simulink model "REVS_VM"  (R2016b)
settings: Solver=ode3  StartTime=REVS.sim_start_time_secs  StopTime=Inf  FixedStep=REVS.sim_step_time_secs  MaxStep=REVS.sim_step_time_secs  EnableMultiTasking=on
StopFcn:
  | postproc_datalog;
  | postproc_audit;
  | postproc_result;
model workspace (MATLAB code in the model file):
  other statements: REVS_setup_variants
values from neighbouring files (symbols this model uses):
  accessory = class_accessory_data    [class_test_data.m]
  battery = class_battery_data    [class_accessory_data.m]    (also in class_REVS_electric.m = class_REVS_battery)
  brake = struct(	'max_torque_Nm',[], 						'proportion_norm',1.0, 						'inertia_kgm2',0.0)    [class_REVS_drive_axle.m]
  engine = class_engine_data    [class_test_data.m]
  final_drive = struct(	'gear_ratio',[], 								'efficiency_norm',[], 								'inertia_kgm2',[] )    [class_REVS_drive_axle.m]
  gear = class_REVS_gearbox    [class_REVS_AT_transmission.m]
  tire = struct(	'radius_m',[], 						'rolling_resistance_coefficient',0, 						'vehicle_weight_norm',1.0,  						'wheel_slip_torque_Nm',[],  						'inertia_kgm2',0.0)    [class_REVS_drive_axle.m]
  torque_converter = class_REVS_torque_converter    [class_REVS_AT_transmission.m]
  transmission = class_transmission_data    [class_test_data.m]
  vehicle = class_vehicle_data    [class_test_data.m]
undefined symbols (not defined in the file or in its folder): alternator, ambient, controls, convert, DelayTimeSecs, drive_cycle, driver, electric, gear_strategy, InitialCondition, InitialValue, LoadSource, LookupStructure, MultiplyPosInputs, Normalize, NumPhases, REVS, SpeedSource, starter, tableshift, UpperSaturationLimit, Value, VerboseLevel, VerboseSignal
libraries: simulink x153
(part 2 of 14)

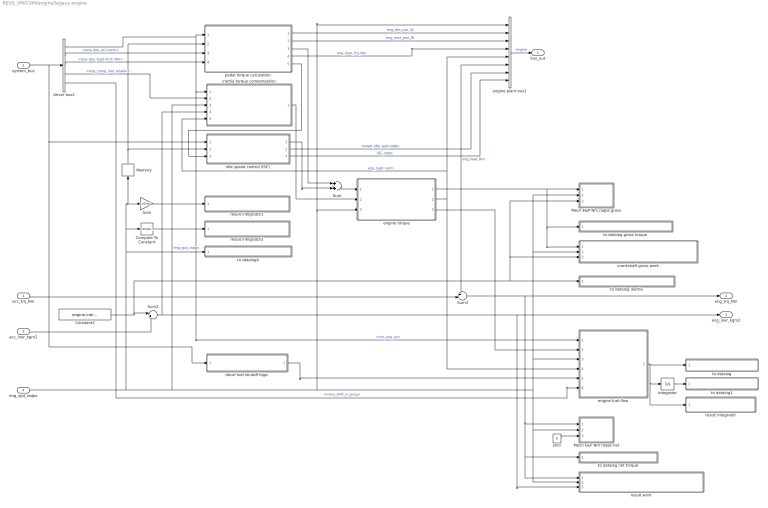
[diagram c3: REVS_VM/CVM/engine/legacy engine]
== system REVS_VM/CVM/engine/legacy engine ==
  system_bus : Inport
  acc_trq_Nm : Inport  Port=2
  acc_iner_kgm2 : Inport  Port=3
  eng_spd_radps : Inport  Port=4
  Compare To Constant : simulink/Logic and Bit Operations/Compare To Constant  relop=>  const=0  OutDataTypeStr=boolean  ZeroCross=off
  Constant2 : Constant  Value=engine.inertia_kgm2
  Gain : Gain  Gain=1/(2*pi)
  Integrator : Integrator
  Mech E&P Nm radps gross : Subsystem
  Mech E&P Nm radps net : Subsystem
  Memory : Memory
  Sum : Sum
  Sum2 : Sum  Inputs=|++
  Sum3 : Sum  Inputs=++|
  crankshaft gross work : Subsystem
  decel fuel shutoff logic : Subsystem
  driver bus2 : BusSelector  OutputSignals=powertrain.control.ctrl_eng_on,powertrain.trans.ctrl.eng_des_acl_norm,powertrain.trans.ctrl.eng_des_load_limit_Nm,powertrain.trans.ctrl.eng_comp_iner_enable,powertrain.trans.ctrl.core_ctl.trans_shift_in_prog
  engine fuel-flow : Subsystem
  engine plant bus1 : BusCreator  Inputs=8
  engine torque : Subsystem
  idle speed control (ISC) : Subsystem
  inertia torque compensation : Subsystem
  pedal torque calculation : Subsystem
  result integrator : Subsystem
  result integrator1 : Subsystem
  result integrator2 : Subsystem
  result work : Subsystem
  to datalog : Subsystem
  to datalog gross torque : Subsystem
  to datalog inertia : Subsystem
  to datalog net torque : Subsystem
  to datalog1 : Subsystem
  to datalog4 : Subsystem
  zero : Constant  Value=0
  bus_out : Outport
  eng_trq_Nm : Outport  Port=2
  eng_iner_kgm2 : Outport  Port=3
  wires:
  idle speed control (ISC)/3(ISC_state) -> engine plant bus1/8  "ISC_state"
  pedal torque calculation/5(current_min_trq_Nm) -> idle speed control (ISC)/3(eng_min_trq_Nm)
  Compare To Constant/1 -> result integrator2/1(in)
  Gain/1 -> result integrator1/1(in)
  driver bus2/5 -> engine fuel-flow/6(shift_in_prog)  "<trans_shift_in_prog>"
  Constant2/1 -> Sum2/1, crankshaft gross work/3(upstream_iner_kgm2), Mech E&P Nm radps gross/3(iner_kgm2), to datalog inertia/1(Var)
  zero/1 -> Mech E&P Nm radps net/3(iner_kgm2)
  eng_spd_radps/1 -> result work/2(speed_radps), Mech E&P Nm radps net/2(spd_radps), Mech E&P Nm radps gross/2(spd_radps), crankshaft gross work/2(speed_radps), engine fuel-flow/3(eng_spd_radps), engine torque/3(eng_spd_radps), engine plant bus1/1, inertia torque compensation/3(eng_spd_radps), to datalog4/1(Var), Compare To Constant/1, Gain/1, Memory/1  "eng_spd_radps"
  Sum3/1 -> eng_trq_Nm/1, Mech E&P Nm radps net/1(" trq_Nm"), to datalog net torque/1(Var), result work/1(torque_Nm)
  engine torque/1(eng_load_Nm) -> Mech E&P Nm radps gross/1(" trq_Nm"), to datalog gross torque/1(Var), crankshaft gross work/1(torque_Nm), Sum3/1, engine plant bus1/6  "eng_load_Nm"
  Integrator/1 -> to datalog1/1(Var)
  engine fuel-flow/1(fuel_flow_rate_gps) -> to datalog/1(Var), Integrator/1, result integrator/1(in)
  inertia torque compensation/1(comp_trq_Nm) -> engine torque/2(eng_fast_trq_Nm)
  pedal torque calculation/4(current_max_trq_Nm) -> engine plant bus1/4  "eng_max_trq_Nm"
  driver bus2/3 -> pedal torque calculation/4(eng_des_load_limit_Nm)  "<eng_des_load_limit_Nm>"
  driver bus2/4 -> inertia torque compensation/2(comp_iner_enable)  "<eng_comp_iner_enable>"
  Sum2/1 -> inertia torque compensation/4(iner_kgm2), eng_iner_kgm2/1, result work/3(upstream_iner_kgm2)
  engine torque/2(eng_load_norm) -> inertia torque compensation/5(load_norm), engine plant bus1/5, engine fuel-flow/4(eng_load_norm)  "eng_load_norm"
  Memory/1 -> idle speed control (ISC)/2(eng_spd_radps), pedal torque calculation/2(eng_spd_radps)
  driver bus2/1 -> pedal torque calculation/1(eng_on), engine fuel-flow/1(eng_on), inertia torque compensation/1(eng_on)  "<ctrl_eng_on>"
  system_bus/1 -> driver bus2/1, idle speed control (ISC)/1(system_bus), decel fuel shutoff logic/1(system_bus)
  Sum/1 -> engine torque/1(eng_slow_trq_Nm)
  idle speed control (ISC)/1(trq_out_Nm) -> Sum/2
  pedal torque calculation/3(des_trq_Nm) -> Sum/1
  engine plant bus1/1 -> bus_out/1  "engine"
  driver bus2/2 -> pedal torque calculation/3(eng_des_acl_norm)  "<eng_des_acl_norm>"
  acc_iner_kgm2/1 -> Sum2/2
  pedal torque calculation/1(des_pwr_W) -> engine plant bus1/2  "eng_des_pwr_W"
  pedal torque calculation/2(current_max_pwr_W) -> engine plant bus1/3  "eng_max_pwr_W"
  acc_trq_Nm/1 -> Sum3/2
  engine torque/3(eng_fuel_trq_Nm) -> engine fuel-flow/2(eng_trq_Nm)
  decel fuel shutoff logic/1(eng_decel_fuel_cut_disable) -> engine fuel-flow/5(eng_decel_fuel_cut_disable)
  idle speed control (ISC)/2(target_idle_spd_radps) -> engine plant bus1/7  "target_idle_spd_radps"

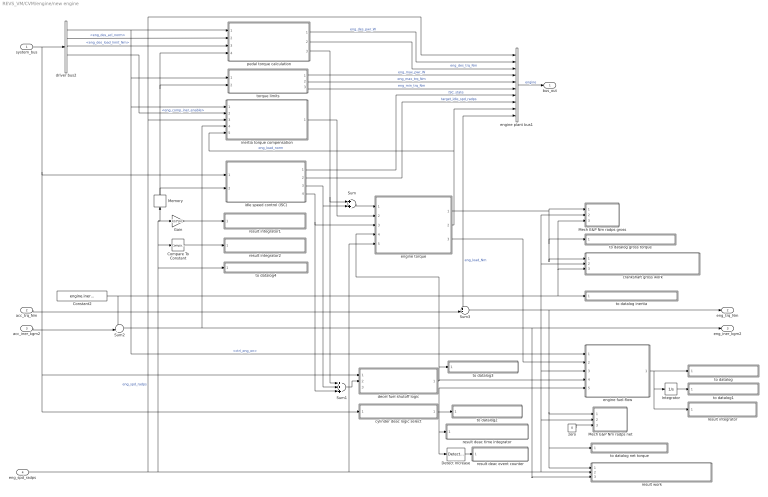
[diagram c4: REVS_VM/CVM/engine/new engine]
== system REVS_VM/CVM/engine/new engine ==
  system_bus : Inport
  acc_trq_Nm : Inport  Port=2
  acc_iner_kgm2 : Inport  Port=3
  eng_spd_radps : Inport  Port=4
  Compare To Constant : simulink/Logic and Bit Operations/Compare To Constant  relop=>  const=0  OutDataTypeStr=boolean  ZeroCross=off
  Constant2 : Constant  Value=engine.inertia_kgm2
  Detect Increase : simulink/Logic and Bit Operations/Detect Increase  vinit=0.0  InputProcessing=Inherited  OutDataTypeStr=boolean
  Gain : Gain  Gain=1/(2*pi)
  Integrator : Integrator
  Mech E&P Nm radps gross : Subsystem
  Mech E&P Nm radps net : Subsystem
  Memory : Memory
  Sum : Sum
  Sum1 : Sum  Inputs=+++
  Sum2 : Sum  Inputs=++|
  Sum3 : Sum  Inputs=++|
  crankshaft gross work : Subsystem
  cylinder deac logic select : Subsystem  Variant=on
  decel fuel shutoff logic : Subsystem
  driver bus2 : BusSelector  OutputSignals=powertrain.control.ctrl_eng_on,powertrain.trans.ctrl.eng_des_acl_norm,powertrain.trans.ctrl.eng_des_load_limit_Nm,powertrain.trans.ctrl.eng_comp_iner_enable,powertrain.trans.ctrl.trans_shift_in_prog
  engine fuel-flow : Subsystem
  engine plant bus1 : BusCreator  Inputs=10
  engine torque : Subsystem
  idle speed control (ISC) : Subsystem
  inertia torque compensation : Subsystem
  pedal torque calculation : Subsystem
  result deac event counter : Subsystem
  result deac time integrator : Subsystem
  result integrator : Subsystem
  result integrator1 : Subsystem
  result integrator2 : Subsystem
  result work : Subsystem
  to datalog : Subsystem
  to datalog gross torque : Subsystem
  to datalog inertia : Subsystem
  to datalog net torque : Subsystem
  to datalog1 : Subsystem
  to datalog2 : Subsystem
  to datalog3 : Subsystem
  to datalog4 : Subsystem
  torque limits : Subsystem
  zero : Constant  Value=0
  bus_out : Outport
  eng_trq_Nm : Outport  Port=2
  eng_iner_kgm2 : Outport  Port=3
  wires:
  decel fuel shutoff logic/1(dfco_active_bool) -> to datalog3/1(Var), engine torque/4(dfco_active_bool), engine fuel-flow/4(eng_decel_fuel_cut_bool)
  Detect Increase/1 -> result deac event counter/1(in)
  cylinder deac logic select/1(cyl_deac_norm) -> result deac time integrator/1(in), Detect Increase/1, to datalog2/1(Var), engine fuel-flow/5(eng_cyl_deac_norm)
  Sum1/1 -> decel fuel shutoff logic/2(eng_rqst_torque_Nm)
  torque limits/3(current_min_trq_Nm) -> engine plant bus1/6  "eng_min_trq_Nm"
  pedal torque calculation/3(des_gross_trq_Nm) -> Sum/1, Sum1/1
  idle speed control (ISC)/4("ISC_fast_trq_Nm ") -> engine torque/3(eng_idle_fast_trq_Nm), Sum1/3
  idle speed control (ISC)/2(ISC_target_spd_radps) -> engine plant bus1/8  "target_idle_spd_radps"
  engine torque/3(eng_fuel_trq_Nm) -> engine fuel-flow/2(eng_trq_Nm)
  acc_trq_Nm/1 -> Sum3/2
  torque limits/1(current_max_pwr_W) -> engine plant bus1/4  "eng_max_pwr_W"
  pedal torque calculation/1(des_pwr_W) -> engine plant bus1/2  "eng_des_pwr_W"
  acc_iner_kgm2/1 -> Sum2/2
  driver bus2/2 -> pedal torque calculation/2(eng_des_acl_norm)  "<eng_des_acl_norm>"
  engine plant bus1/1 -> bus_out/1  "engine"
  pedal torque calculation/2(des_trq_Nm) -> engine plant bus1/3  "eng_des_trq_Nm"
  idle speed control (ISC)/3(ISC_slow_trq_Nm) -> Sum/2, Sum1/2
  Sum/1 -> engine torque/1(eng_slow_trq_Nm)
  system_bus/1 -> driver bus2/1, idle speed control (ISC)/1(system_bus), decel fuel shutoff logic/1(system_bus), cylinder deac logic select/1(system_bus)
  driver bus2/1 -> engine fuel-flow/1(eng_on), inertia torque compensation/1(eng_on), torque limits/1(eng_on), pedal torque calculation/1(eng_on)  "<ctrl_eng_on>"
  Memory/1 -> idle speed control (ISC)/2(eng_spd_radps), torque limits/2(eng_spd_radps), pedal torque calculation/4(eng_spd_radps)
  engine torque/2(eng_load_norm) -> inertia torque compensation/5(load_norm), engine plant bus1/9  "eng_load_norm"
  Sum2/1 -> result work/3(upstream_iner_kgm2), eng_iner_kgm2/1, inertia torque compensation/4(iner_kgm2)
  driver bus2/4 -> inertia torque compensation/2(comp_iner_enable)  "<eng_comp_iner_enable>"
  driver bus2/3 -> pedal torque calculation/3(eng_des_load_limit_Nm)  "<eng_des_load_limit_Nm>"
  torque limits/2(current_max_trq_Nm) -> engine plant bus1/5  "eng_max_trq_Nm"
  inertia torque compensation/1(comp_trq_Nm) -> engine torque/2(eng_fast_trq_Nm)
  engine fuel-flow/1(fuel_flow_rate_gps) -> result integrator/1(in), Integrator/1, to datalog/1(Var)
  Integrator/1 -> to datalog1/1(Var)
  engine torque/1(eng_load_Nm) -> crankshaft gross work/1(torque_Nm), to datalog gross torque/1(Var), Mech E&P Nm radps gross/1(" trq_Nm"), engine plant bus1/10, Sum3/1  "eng_load_Nm"
  Sum3/1 -> to datalog net torque/1(Var), result work/1(torque_Nm), Mech E&P Nm radps net/1(" trq_Nm"), eng_trq_Nm/1
  eng_spd_radps/1 -> result work/2(speed_radps), engine fuel-flow/3(eng_spd_radps), crankshaft gross work/2(speed_radps), Mech E&P Nm radps gross/2(spd_radps), Mech E&P Nm radps net/2(spd_radps), engine torque/5(eng_spd_radps), to datalog4/1(Var), Compare To Constant/1, Gain/1, Memory/1, inertia torque compensation/3(eng_spd_radps), engine plant bus1/1  "eng_spd_radps"
  zero/1 -> Mech E&P Nm radps net/3(iner_kgm2)
  Constant2/1 -> Sum2/1, Mech E&P Nm radps gross/3(iner_kgm2), crankshaft gross work/3(upstream_iner_kgm2), to datalog inertia/1(Var)
  Gain/1 -> result integrator1/1(in)
  Compare To Constant/1 -> result integrator2/1(in)
  idle speed control (ISC)/1(ISC_state) -> engine plant bus1/7  "ISC_state"

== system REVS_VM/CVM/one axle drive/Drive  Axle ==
  system bus : Inport
  trq_in_Nm : Inport  Port=2
  iner_in_kgm2 : Inport  Port=3
  spd_out_mps : Inport  Port=4
  Sum : Sum
  Sum1 : Sum
  brakes : Subsystem
  final drive : Subsystem
  result work : Subsystem
  tires : Subsystem
  to datalog : Subsystem
  to datalog1 : Subsystem
  to datalog2 : Subsystem
  force_out_N : Outport
  mass_out_kg : Outport  Port=2
  spd_in_radps : Outport  Port=3
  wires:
  final drive/3(spd_in_radps) -> spd_in_radps/1
  final drive/2(iner_out_kgm2) -> Sum1/2, to datalog1/1(Var), result work/3(upstream_iner_kgm2)
  final drive/1(trq_out_Nm) -> brakes/2(trq_in_Nm), Sum/2, to datalog/1(Var), result work/1(torque_Nm)
  iner_in_kgm2/1 -> final drive/2(iner_in_kgm2)
  trq_in_Nm/1 -> final drive/1(trq_in_Nm)
  brakes/2(iner_out_kgm2) -> Sum1/1
  Sum1/1 -> tires/3(iner_in_kgm2)
  brakes/1(trq_out_Nm) -> Sum/1
  Sum/1 -> tires/2(trq_in_Nm)
  system bus/1 -> brakes/1(system_bus), tires/1(system_bus)
  spd_out_mps/1 -> tires/4(spd_out_mps)
  tires/3(spd_in_radps) -> brakes/3(spd_in_radps), final drive/3(spd_out_radps), to datalog2/1(Var), result work/2(speed_radps)
  tires/1(force_out_N) -> force_out_N/1
  tires/2(mass_out_kg) -> mass_out_kg/1

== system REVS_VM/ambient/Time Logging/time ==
  "time " : Inport
  Enable : EnablePort
  To Workspace : ToWorkspace  VariableName=time  SampleTime=-1
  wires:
  "time "/1 -> To Workspace/1

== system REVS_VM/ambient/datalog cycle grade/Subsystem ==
  In1 : Inport
  Enable : EnablePort
  To Workspace : ToWorkspace  VariableName=datalog__drive_cycle_grade_pct  SampleTime=-1
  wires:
  In1/1 -> To Workspace/1

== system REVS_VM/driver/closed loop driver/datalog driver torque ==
  Var : Inport
  Constant : Constant  Value=VerboseSignal
  Constant1 : Constant  Value=VerboseLevel
  Relational Operator : RelationalOperator  OutDataTypeStr=boolean  ZeroCross=off
  Subsystem : Subsystem
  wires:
  Constant1/1 -> Relational Operator/2
  Constant/1 -> Relational Operator/1
  Relational Operator/1 -> Subsystem/Enable
  Var/1 -> Subsystem/1(In1)

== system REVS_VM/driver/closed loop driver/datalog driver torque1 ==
  Var : Inport
  Constant : Constant  Value=VerboseSignal
  Constant1 : Constant  Value=VerboseLevel
  Relational Operator : RelationalOperator  OutDataTypeStr=boolean  ZeroCross=off
  Subsystem : Subsystem
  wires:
  Constant1/1 -> Relational Operator/2
  Constant/1 -> Relational Operator/1
  Relational Operator/1 -> Subsystem/Enable
  Var/1 -> Subsystem/1(In1)

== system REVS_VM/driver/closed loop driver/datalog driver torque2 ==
  Var : Inport
  Constant : Constant  Value=VerboseSignal
  Constant1 : Constant  Value=VerboseLevel
  Relational Operator : RelationalOperator  OutDataTypeStr=boolean  ZeroCross=off
  Subsystem : Subsystem
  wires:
  Constant1/1 -> Relational Operator/2
  Constant/1 -> Relational Operator/1
  Relational Operator/1 -> Subsystem/Enable
  Var/1 -> Subsystem/1(In1)

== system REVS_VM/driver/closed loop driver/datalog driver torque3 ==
  Var : Inport
  Constant : Constant  Value=VerboseSignal
  Constant1 : Constant  Value=VerboseLevel
  Relational Operator : RelationalOperator  OutDataTypeStr=boolean  ZeroCross=off
  Subsystem : Subsystem
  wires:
  Constant1/1 -> Relational Operator/2
  Constant/1 -> Relational Operator/1
  Relational Operator/1 -> Subsystem/Enable
  Var/1 -> Subsystem/1(In1)

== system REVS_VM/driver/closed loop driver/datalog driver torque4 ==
  Var : Inport
  Constant : Constant  Value=VerboseSignal
  Constant1 : Constant  Value=VerboseLevel
  Relational Operator : RelationalOperator  OutDataTypeStr=boolean  ZeroCross=off
  Subsystem : Subsystem
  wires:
  Constant1/1 -> Relational Operator/2
  Constant/1 -> Relational Operator/1
  Relational Operator/1 -> Subsystem/Enable
  Var/1 -> Subsystem/1(In1)

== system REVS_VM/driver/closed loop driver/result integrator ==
  in : Inport
  Data Type Conversion : DataTypeConversion  OutDataTypeStr=double
  Integrator1 : Integrator  UpperSaturationLimit=Inf  LowerSaturationLimit=0  ZeroCross=off
  Integrator2 : Integrator  UpperSaturationLimit=Inf  LowerSaturationLimit=0  ZeroCross=off
  Phase To Workspace : ToWorkspace  VariableName=result__phase_driver_error_time_secs  SampleTime=-1
  Product1 : Product  Multiplication=Matrix(*)
  Reshape : Reshape
  Total To Workspace : ToWorkspace  VariableName=result__total_driver_error_time_secs  SampleTime=-1
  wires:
  Reshape/1 -> Integrator1/1, Product1/1
  Data Type Conversion/1 -> Reshape/1
  Integrator2/1 -> Phase To Workspace/1
  [REVS_phase_flag] -> Product1/2
  Product1/1 -> Integrator2/1
  Integrator1/1 -> Total To Workspace/1
  in/1 -> Data Type Conversion/1

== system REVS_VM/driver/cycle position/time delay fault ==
  " condition" : Inport
  Assertion : Assertion  AssertionFailFcn=error('Klaatu Berada Nicto')
  Compare To Constant1 : simulink/Logic and Bit Operations/Compare To Constant  relop=<  const=DelayTimeSecs  OutDataTypeStr=boolean  ZeroCross=off
  Compare To Constant2 : simulink/Logic and Bit Operations/Compare To Constant  relop=>  const=DelayTimeSecs + 0.1  OutDataTypeStr=boolean  ZeroCross=off
  Data Type Conversion : DataTypeConversion
  Integrator1 : Integrator  ExternalReset=falling  ZeroCross=off
  Stop Simulation : Stop
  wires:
  Compare To Constant2/1 -> Stop Simulation/1
  Data Type Conversion/1 -> Integrator1/1, Integrator1/2
  Integrator1/1 -> Compare To Constant1/1, Compare To Constant2/1
  " condition"/1 -> Data Type Conversion/1
  Compare To Constant1/1 -> Assertion/1

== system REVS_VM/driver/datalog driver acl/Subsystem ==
  In1 : Inport
  Enable : EnablePort
  To Workspace : ToWorkspace  VariableName=datalog__driver__accel_norm  SampleTime=-1
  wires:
  In1/1 -> To Workspace/1

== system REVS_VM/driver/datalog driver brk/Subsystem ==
  In1 : Inport
  Enable : EnablePort
  To Workspace : ToWorkspace  VariableName=datalog__driver__brake_norm  SampleTime=-1
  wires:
  In1/1 -> To Workspace/1

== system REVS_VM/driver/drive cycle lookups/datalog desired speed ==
  Var : Inport
  Constant : Constant  Value=VerboseSignal
  Constant1 : Constant  Value=VerboseLevel
  Relational Operator : RelationalOperator  OutDataTypeStr=boolean  ZeroCross=off
  Subsystem : Subsystem
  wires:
  Constant1/1 -> Relational Operator/2
  Constant/1 -> Relational Operator/1
  Relational Operator/1 -> Subsystem/Enable
  Var/1 -> Subsystem/1(In1)

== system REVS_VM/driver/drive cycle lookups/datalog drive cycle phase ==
  Var : Inport
  Constant : Constant  Value=VerboseSignal
  Constant1 : Constant  Value=VerboseLevel
  Relational Operator : RelationalOperator  OutDataTypeStr=boolean  ZeroCross=off
  Subsystem : Subsystem
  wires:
  Constant1/1 -> Relational Operator/2
  Constant/1 -> Relational Operator/1
  Relational Operator/1 -> Subsystem/Enable
  Var/1 -> Subsystem/1(In1)

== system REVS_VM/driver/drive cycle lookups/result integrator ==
  in : Inport
  Data Type Conversion : DataTypeConversion  OutDataTypeStr=double
  Integrator1 : Integrator  UpperSaturationLimit=Inf  LowerSaturationLimit=0  ZeroCross=off
  Integrator2 : Integrator  UpperSaturationLimit=Inf  LowerSaturationLimit=0  ZeroCross=off
  Phase To Workspace : ToWorkspace  VariableName=result__phase_drive_cycle_distance_m  SampleTime=-1
  Product1 : Product  Multiplication=Matrix(*)
  Reshape : Reshape
  Total To Workspace : ToWorkspace  VariableName=result__total_drive_cycle_distance_m  SampleTime=-1
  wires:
  Reshape/1 -> Integrator1/1, Product1/1
  Data Type Conversion/1 -> Reshape/1
  Integrator2/1 -> Phase To Workspace/1
  [REVS_phase_flag] -> Product1/2
  Product1/1 -> Integrator2/1
  Integrator1/1 -> Total To Workspace/1
  in/1 -> Data Type Conversion/1

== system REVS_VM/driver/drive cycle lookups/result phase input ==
  phase : Inport
  Constant : Constant
  Constant1 : Constant  Value=[1:NumPhases]  VectorParams1D=off
  Data Type Conversion : DataTypeConversion
  Display : Display
  Integrator1 : Integrator  UpperSaturationLimit=Inf  LowerSaturationLimit=0  ZeroCross=off
  Integrator2 : Integrator  UpperSaturationLimit=Inf  LowerSaturationLimit=0  ZeroCross=off
  Phase To Workspace : ToWorkspace  VariableName=result__phase_time_secs  SampleTime=-1
  Relational Operator : RelationalOperator  Operator===  OutDataTypeStr=boolean  ZeroCross=off
  Signal Specification : SignalSpecification  Dimensions=1
  Total To Workspace : ToWorkspace  VariableName=result__total_time_secs  SampleTime=-1
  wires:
  Signal Specification/1 -> Relational Operator/1
  Data Type Conversion/1 -> Integrator2/1, [REVS_phase_flag], Display/1
  phase/1 -> Signal Specification/1
  Constant1/1 -> Relational Operator/2
  Constant/1 -> Integrator1/1
  Integrator1/1 -> Total To Workspace/1
  Relational Operator/1 -> Data Type Conversion/1
  Integrator2/1 -> Phase To Workspace/1

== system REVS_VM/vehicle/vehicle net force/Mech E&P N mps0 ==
  force_N : Inport
  spd_mps : Inport  Port=2
  Compare To Constant : simulink/Logic and Bit Operations/Compare To Constant  relop=>=  const=1  OutDataTypeStr=boolean
  Constant : Constant  Value=VerboseSignal
  Subsystem : Subsystem
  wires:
  Constant/1 -> Compare To Constant/1
  Compare To Constant/1 -> Subsystem/Enable
  spd_mps/1 -> Subsystem/2(spd_mps)
  force_N/1 -> Subsystem/1(force_N)

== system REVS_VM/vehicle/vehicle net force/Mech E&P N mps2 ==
  force_N : Inport
  spd_mps : Inport  Port=2
  Compare To Constant : simulink/Logic and Bit Operations/Compare To Constant  relop=>=  const=1  OutDataTypeStr=boolean
  Constant : Constant  Value=VerboseSignal
  Subsystem : Subsystem
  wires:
  Constant/1 -> Compare To Constant/1
  Compare To Constant/1 -> Subsystem/Enable
  spd_mps/1 -> Subsystem/2(spd_mps)
  force_N/1 -> Subsystem/1(force_N)

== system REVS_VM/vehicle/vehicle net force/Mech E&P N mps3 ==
  force_N : Inport
  spd_mps : Inport  Port=2
  mass_kg : Inport  Port=3
  Compare To Constant : simulink/Logic and Bit Operations/Compare To Constant  relop=>=  const=1  OutDataTypeStr=boolean
  Constant : Constant  Value=VerboseSignal
  Subsystem : Subsystem
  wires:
  Constant/1 -> Compare To Constant/1
  Compare To Constant/1 -> Subsystem/Enable
  mass_kg/1 -> Subsystem/3(mass_kg)
  spd_mps/1 -> Subsystem/2(spd_mps)
  force_N/1 -> Subsystem/1(force_N)

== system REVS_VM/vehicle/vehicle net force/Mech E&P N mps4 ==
  force_N : Inport
  spd_mps : Inport  Port=2
  Compare To Constant : simulink/Logic and Bit Operations/Compare To Constant  relop=>=  const=1  OutDataTypeStr=boolean
  Constant : Constant  Value=VerboseSignal
  Subsystem : Subsystem
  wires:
  Constant/1 -> Compare To Constant/1
  Compare To Constant/1 -> Subsystem/Enable
  spd_mps/1 -> Subsystem/2(spd_mps)
  force_N/1 -> Subsystem/1(force_N)

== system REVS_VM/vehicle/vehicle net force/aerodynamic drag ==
  veh_spd_mps : Inport
  Aero Drag Force (N) : Product  Inputs=5
  Air Density (kg/m^3) : Constant  Value=ambient.air_density_kgpm3
  Drag Coefficient : Constant  Value=vehicle.aerodynamic_drag_coeff
  Frontal Area (m^2) : Constant  Value=vehicle.frontal_area_m2
  Gain : Gain  Gain=0.5
  Math Function : Math  Operator=square
  Sign : Signum  ZeroCross=off
  aero_force_N : Outport
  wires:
  veh_spd_mps/1 -> Sign/1, Math Function/1
  Sign/1 -> Gain/1
  Aero Drag Force (N)/1 -> aero_force_N/1
  Gain/1 -> Aero Drag Force (N)/2
  Drag Coefficient/1 -> Aero Drag Force (N)/5
  Frontal Area (m^2)/1 -> Aero Drag Force (N)/4
  Air Density (kg/m^3)/1 -> Aero Drag Force (N)/3
  Math Function/1 -> Aero Drag Force (N)/1

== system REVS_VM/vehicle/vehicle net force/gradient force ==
  system_bus : Inport
  % grade to norm : Gain  Gain=0.01
  Bus Selector : BusSelector  OutputSignals=ambient.drive_cycle_grade_pct
  Gradient Force (N) : Product  Inputs=3
  Gravitational Acceleration (m/sec^2) : Constant  Value=ambient.gravity_mps2
  Static Vehicle Mass (kg) : Constant  Value=vehicle.mass_static_kg
  Sum : Sum  Inputs=|++
  Trigonometric Function : Trigonometry  Operator=atan
  Trigonometric Function1 : Trigonometry
  dynamic lookup : Subsystem
  grade_force_N : Outport
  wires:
  Static Vehicle Mass (kg)/1 -> Sum/2
  dynamic lookup/1(out) -> Sum/1
  Sum/1 -> Gradient Force (N)/3
  system_bus/1 -> Bus Selector/1, dynamic lookup/1(bus)
  Bus Selector/1 -> % grade to norm/1  "<drive_cycle_grade_pct>"
  Gravitational Acceleration (m/sec^2)/1 -> Gradient Force (N)/2
  Trigonometric Function/1 -> Trigonometric Function1/1
  % grade to norm/1 -> Trigonometric Function/1
  Gradient Force (N)/1 -> grade_force_N/1
  Trigonometric Function1/1 -> Gradient Force (N)/1

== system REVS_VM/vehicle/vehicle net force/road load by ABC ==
  system_bus : Inport
  veh_spd_mps : Inport  Port=2
  Abs : Abs
  B-Term : Product
  B-Term1 : Product  Inputs=*/
  B-Term2 : Product
  C-Term : Product
  Coastdown Coefficient A : Constant  Value=vehicle.coastdown_target_A_N + vehicle.coastdown_adjust_A_N
  Coastdown Coefficient B : Constant  Value=vehicle.coastdown_target_B_Npms + vehicle.coastdown_adjust_B_Npms
  Coastdown Coefficient C : Constant  Value=vehicle.coastdown_target_C_Npms2 + vehicle.coastdown_adjust_C_Npms2
  Math Function : Math  Operator=square
  Road Load (N) : Sum  Inputs=+++
  Sign : Product
  Static Vehicle Mass (kg) : Constant  Value=vehicle.mass_static_kg
  Sum : Sum  Inputs=|++
  dynamic lookup : Subsystem
  sign : Lookup_n-D  NumberOfTableDimensions=1  BreakpointsForDimension1=[-eps 0 eps]  BeginIndexSearchUsingPreviousIndexResult=on  Table=[-1 1 1]  ExtrapMethod=Clip  UseLastTableValue=on  RndMeth=Simplest
  rdload_force_N : Outport
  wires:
  B-Term2/1 -> Road Load (N)/1
  B-Term1/1 -> B-Term2/1
  Coastdown Coefficient A/1 -> B-Term2/2
  Sum/1 -> B-Term1/1
  Static Vehicle Mass (kg)/1 -> Sum/2, B-Term1/2
  dynamic lookup/1(out) -> Sum/1
  system_bus/1 -> dynamic lookup/1(bus)
  sign/1 -> Sign/2
  Abs/1 -> B-Term/1
  Math Function/1 -> C-Term/1
  veh_spd_mps/1 -> Math Function/1, sign/1, Abs/1
  Coastdown Coefficient B/1 -> B-Term/2
  C-Term/1 -> Road Load (N)/3
  Sign/1 -> rdload_force_N/1
  B-Term/1 -> Road Load (N)/2
  Coastdown Coefficient C/1 -> C-Term/2
  Road Load (N)/1 -> Sign/1

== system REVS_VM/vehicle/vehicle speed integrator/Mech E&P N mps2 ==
  force_N : Inport
  spd_mps : Inport  Port=2
  mass_kg : Inport  Port=3
  Compare To Constant : simulink/Logic and Bit Operations/Compare To Constant  relop=>=  const=1  OutDataTypeStr=boolean
  Constant : Constant  Value=VerboseSignal
  Subsystem : Subsystem
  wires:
  Constant/1 -> Compare To Constant/1
  Compare To Constant/1 -> Subsystem/Enable
  mass_kg/1 -> Subsystem/3(mass_kg)
  spd_mps/1 -> Subsystem/2(spd_mps)
  force_N/1 -> Subsystem/1(force_N)

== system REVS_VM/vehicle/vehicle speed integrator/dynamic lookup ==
  bus : Inport
  Bus Selector : BusSelector  OutputSignals=gb.gb_cmd_gear,gb_spd_in_radps,ctrl.gb_line_press_bar
  Lookup : Lookup_n-D  NumberOfTableDimensions=10  BreakpointsForDimension1=LookupStructure.axis_1.breakpoints  BreakpointsForDimension2=LookupStructure.axis_2.breakpoints  BreakpointsForDimension3=LookupStructure.axis_3.breakpoints  BreakpointsForDimension4=LookupStructure.axis_4.breakpoints  BreakpointsForDimension5=LookupStructure.axis_5.breakpoints  BreakpointsForDimension6=LookupStructure.axis_6.breakpoints  BreakpointsForDimension7=LookupStructure.axis_7.breakpoints  BreakpointsForDimension8=LookupStructure.axis_8.breakpoints  BreakpointsForDimension9=LookupStructure.axis_9.breakpoints  BreakpointsForDimension10=LookupStructure.axis_10.breakpoints  IndexSearchMethod=Linear search  BeginIndexSearchUsingPreviousIndexResult=on  Table=LookupStructure.table  DiagnosticForOutOfRangeInput=Warning  InternalRulePriority=Speed  RndMeth=Simplest  SupportTunableTableSize=on  MaximumIndicesForEachDimension=LookupStructure.table_size
  out : Outport
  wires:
  bus/1 -> Bus Selector/1
  Lookup/1 -> out/1

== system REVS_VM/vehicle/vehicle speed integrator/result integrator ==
  in : Inport
  Data Type Conversion : DataTypeConversion  OutDataTypeStr=double
  Integrator1 : Integrator  UpperSaturationLimit=Inf  LowerSaturationLimit=0  ZeroCross=off
  Integrator2 : Integrator  UpperSaturationLimit=Inf  LowerSaturationLimit=0  ZeroCross=off
  Phase To Workspace : ToWorkspace  VariableName=result__phase_distance_m  SampleTime=-1
  Product1 : Product  Multiplication=Matrix(*)
  Reshape : Reshape
  Total To Workspace : ToWorkspace  VariableName=result__total_distance_m  SampleTime=-1
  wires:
  Reshape/1 -> Integrator1/1, Product1/1
  Data Type Conversion/1 -> Reshape/1
  Integrator2/1 -> Phase To Workspace/1
  [REVS_phase_flag] -> Product1/2
  Product1/1 -> Integrator2/1
  Integrator1/1 -> Total To Workspace/1
  in/1 -> Data Type Conversion/1

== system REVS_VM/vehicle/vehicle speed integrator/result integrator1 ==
  in : Inport
  Data Type Conversion : DataTypeConversion  OutDataTypeStr=double
  Integrator1 : Integrator  UpperSaturationLimit=Inf  LowerSaturationLimit=0  ZeroCross=off
  Integrator2 : Integrator  UpperSaturationLimit=Inf  LowerSaturationLimit=0  ZeroCross=off
  Phase To Workspace : ToWorkspace  VariableName=result__phase_stopped_time_secs  SampleTime=-1
  Product1 : Product  Multiplication=Matrix(*)
  Reshape : Reshape
  Total To Workspace : ToWorkspace  VariableName=result__total_stopped_time_secs  SampleTime=-1
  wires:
  Reshape/1 -> Integrator1/1, Product1/1
  Data Type Conversion/1 -> Reshape/1
  Integrator2/1 -> Phase To Workspace/1
  [REVS_phase_flag] -> Product1/2
  Product1/1 -> Integrator2/1
  Integrator1/1 -> Total To Workspace/1
  in/1 -> Data Type Conversion/1

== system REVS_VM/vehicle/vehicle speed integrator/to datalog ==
  Var : Inport
  Constant : Constant  Value=VerboseSignal
  Constant1 : Constant  Value=VerboseLevel
  Relational Operator : RelationalOperator  OutDataTypeStr=boolean  ZeroCross=off
  Subsystem : Subsystem
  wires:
  Constant1/1 -> Relational Operator/2
  Constant/1 -> Relational Operator/1
  Relational Operator/1 -> Subsystem/Enable
  Var/1 -> Subsystem/1(In1)

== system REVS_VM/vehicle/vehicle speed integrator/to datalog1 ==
  Var : Inport
  Constant : Constant  Value=VerboseSignal
  Constant1 : Constant  Value=VerboseLevel
  Relational Operator : RelationalOperator  OutDataTypeStr=boolean  ZeroCross=off
  Subsystem : Subsystem
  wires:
  Constant1/1 -> Relational Operator/2
  Constant/1 -> Relational Operator/1
  Relational Operator/1 -> Subsystem/Enable
  Var/1 -> Subsystem/1(In1)

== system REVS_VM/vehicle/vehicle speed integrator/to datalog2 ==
  Var : Inport
  Constant : Constant  Value=VerboseSignal
  Constant1 : Constant  Value=VerboseLevel
  Relational Operator : RelationalOperator  OutDataTypeStr=boolean  ZeroCross=off
  Subsystem : Subsystem
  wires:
  Constant1/1 -> Relational Operator/2
  Constant/1 -> Relational Operator/1
  Relational Operator/1 -> Subsystem/Enable
  Var/1 -> Subsystem/1(In1)

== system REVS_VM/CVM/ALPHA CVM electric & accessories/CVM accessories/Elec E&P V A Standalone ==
  volts_V : Inport
  curr_A : Inport  Port=2
  Compare To Constant : simulink/Logic and Bit Operations/Compare To Constant  relop=>=  const=1  OutDataTypeStr=boolean
  Constant : Constant  Value=VerboseSignal
  Subsystem : Subsystem
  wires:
  Constant/1 -> Compare To Constant/1
  Compare To Constant/1 -> Subsystem/Enable
  curr_A/1 -> Subsystem/2(curr_A)
  volts_V/1 -> Subsystem/1(volts_V)

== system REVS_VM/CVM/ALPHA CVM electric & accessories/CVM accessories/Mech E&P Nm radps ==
  trq_Nm : Inport
  spd_radps : Inport  Port=2
  Compare To Constant : simulink/Logic and Bit Operations/Compare To Constant  relop=>=  const=1  OutDataTypeStr=boolean
  Constant : Constant  Value=VerboseSignal
  Subsystem : Subsystem
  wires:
  Constant/1 -> Compare To Constant/1
  Compare To Constant/1 -> Subsystem/Enable
  spd_radps/1 -> Subsystem/2(spd_radps)
  trq_Nm/1 -> Subsystem/1(trq_Nm)

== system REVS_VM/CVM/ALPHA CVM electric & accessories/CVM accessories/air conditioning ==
  system_bus : Inport
  voltage_volts : Inport  Port=2
  speed_radps : Inport  Port=3
  Bus Creator : BusCreator  Inputs=3
  Bus Selector : BusSelector  OutputSignals=driver.driver_ign_keyon
  Elec E&P V A Standalone : Subsystem
  Gain : Gain  Gain=-1
  Mech E&P Nm radps : Subsystem
  Product1 : Product  Inputs=**
  Product5 : Product  Inputs=***
  electrical loss map : Subsystem
  mechanical loss map : Subsystem
  rotational inertia : Constant  Value=accessory.inertia_kgm2
  rotational inertia5 : Constant  Value=accessory.enable
  curr_in_A : Outport
  torque_Nm : Outport  Port=2
  inertia_kgm2 : Outport  Port=3
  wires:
  Bus Creator/1 -> electrical loss map/1(bus), mechanical loss map/1(bus)
  Product1/1 -> Gain/1
  Bus Selector/1 -> Product5/2  "<driver_ign_keyon>"
  mechanical loss map/1(out) -> Product1/2
  rotational inertia5/1 -> Product5/1, Product1/1
  electrical loss map/1(out) -> Product5/3
  speed_radps/1 -> Bus Creator/3, Mech E&P Nm radps/2(spd_radps)  "acc_spd_radps"
  rotational inertia/1 -> inertia_kgm2/1, Mech E&P Nm radps/3(iner_kgm2)
  Gain/1 -> torque_Nm/1, Mech E&P Nm radps/1(" trq_Nm")
  Product5/1 -> curr_in_A/1, Elec E&P V A Standalone/2(curr_A)
  voltage_volts/1 -> Bus Creator/2, Elec E&P V A Standalone/1(volts_V)  "acc_volt_V"
  system_bus/1 -> Bus Creator/1, Bus Selector/1  "system_bus"

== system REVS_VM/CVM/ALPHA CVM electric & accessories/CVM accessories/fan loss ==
  system_bus : Inport
  voltage_volts : Inport  Port=2
  speed_radps : Inport  Port=3
  Bus Creator : BusCreator  Inputs=3
  Bus Selector : BusSelector  OutputSignals=driver.driver_ign_keyon
  Elec E&P V A Standalone : Subsystem
  Gain : Gain  Gain=-1
  Mech E&P Nm radps : Subsystem
  Product1 : Product  Inputs=**
  Product5 : Product  Inputs=***
  electrical loss map : Subsystem
  mechanical loss map : Subsystem
  rotational inertia : Constant  Value=accessory.inertia_kgm2
  rotational inertia5 : Constant  Value=accessory.enable
  curr_in_A : Outport
  torque_Nm : Outport  Port=2
  inertia_kgm2 : Outport  Port=3
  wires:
  Bus Creator/1 -> electrical loss map/1(bus), mechanical loss map/1(bus)
  Product1/1 -> Gain/1
  Bus Selector/1 -> Product5/2  "<driver_ign_keyon>"
  mechanical loss map/1(out) -> Product1/2
  rotational inertia5/1 -> Product5/1, Product1/1
  electrical loss map/1(out) -> Product5/3
  speed_radps/1 -> Bus Creator/3, Mech E&P Nm radps/2(spd_radps)  "acc_spd_radps"
  rotational inertia/1 -> inertia_kgm2/1, Mech E&P Nm radps/3(iner_kgm2)
  Gain/1 -> torque_Nm/1, Mech E&P Nm radps/1(" trq_Nm")
  Product5/1 -> curr_in_A/1, Elec E&P V A Standalone/2(curr_A)
  voltage_volts/1 -> Bus Creator/2, Elec E&P V A Standalone/1(volts_V)  "acc_volt_V"
  system_bus/1 -> Bus Creator/1, Bus Selector/1  "system_bus"

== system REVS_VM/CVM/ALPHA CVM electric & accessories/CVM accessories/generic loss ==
  system_bus : Inport
  voltage_volts : Inport  Port=2
  speed_radps : Inport  Port=3
  Bus Creator : BusCreator  Inputs=3
  Bus Selector : BusSelector  OutputSignals=driver.driver_ign_keyon
  Elec E&P V A Standalone : Subsystem
  Gain : Gain  Gain=-1
  Mech E&P Nm radps : Subsystem
  Product1 : Product  Inputs=**
  Product5 : Product  Inputs=***
  electrical loss map : Subsystem
  mechanical loss map : Subsystem
  rotational inertia : Constant  Value=accessory.inertia_kgm2
  rotational inertia5 : Constant  Value=accessory.enable
  curr_in_A : Outport
  torque_Nm : Outport  Port=2
  inertia_kgm2 : Outport  Port=3
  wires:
  Bus Creator/1 -> electrical loss map/1(bus), mechanical loss map/1(bus)
  Product1/1 -> Gain/1
  Bus Selector/1 -> Product5/2  "<driver_ign_keyon>"
  mechanical loss map/1(out) -> Product1/2
  rotational inertia5/1 -> Product5/1, Product1/1
  electrical loss map/1(out) -> Product5/3
  speed_radps/1 -> Bus Creator/3, Mech E&P Nm radps/2(spd_radps)  "acc_spd_radps"
  rotational inertia/1 -> inertia_kgm2/1, Mech E&P Nm radps/3(iner_kgm2)
  Gain/1 -> torque_Nm/1, Mech E&P Nm radps/1(" trq_Nm")
  Product5/1 -> curr_in_A/1, Elec E&P V A Standalone/2(curr_A)
  voltage_volts/1 -> Bus Creator/2, Elec E&P V A Standalone/1(volts_V)  "acc_volt_V"
  system_bus/1 -> Bus Creator/1, Bus Selector/1  "system_bus"

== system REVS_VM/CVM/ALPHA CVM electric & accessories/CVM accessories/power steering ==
  system_bus : Inport
  voltage_volts : Inport  Port=2
  speed_radps : Inport  Port=3
  Bus Creator : BusCreator  Inputs=3
  Bus Selector : BusSelector  OutputSignals=driver.driver_ign_keyon
  Elec E&P V A Standalone : Subsystem
  Gain : Gain  Gain=-1
  Mech E&P Nm radps : Subsystem
  Product1 : Product  Inputs=**
  Product5 : Product  Inputs=***
  electrical loss map : Subsystem
  mechanical loss map : Subsystem
  rotational inertia : Constant  Value=accessory.inertia_kgm2
  rotational inertia5 : Constant  Value=accessory.enable
  curr_in_A : Outport
  torque_Nm : Outport  Port=2
  inertia_kgm2 : Outport  Port=3
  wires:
  Bus Creator/1 -> electrical loss map/1(bus), mechanical loss map/1(bus)
  Product1/1 -> Gain/1
  Bus Selector/1 -> Product5/2  "<driver_ign_keyon>"
  mechanical loss map/1(out) -> Product1/2
  rotational inertia5/1 -> Product5/1, Product1/1
  electrical loss map/1(out) -> Product5/3
  speed_radps/1 -> Bus Creator/3, Mech E&P Nm radps/2(spd_radps)  "acc_spd_radps"
  rotational inertia/1 -> inertia_kgm2/1, Mech E&P Nm radps/3(iner_kgm2)
  Gain/1 -> torque_Nm/1, Mech E&P Nm radps/1(" trq_Nm")
  Product5/1 -> curr_in_A/1, Elec E&P V A Standalone/2(curr_A)
  voltage_volts/1 -> Bus Creator/2, Elec E&P V A Standalone/1(volts_V)  "acc_volt_V"
  system_bus/1 -> Bus Creator/1, Bus Selector/1  "system_bus"

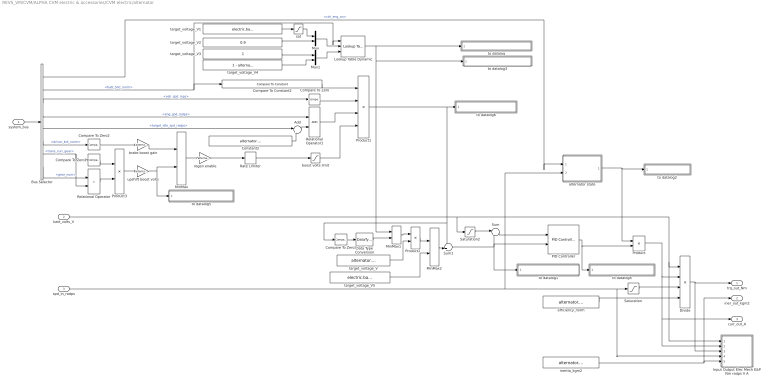
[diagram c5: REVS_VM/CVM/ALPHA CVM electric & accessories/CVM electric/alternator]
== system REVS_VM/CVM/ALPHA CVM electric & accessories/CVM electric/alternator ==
  system_bus : Inport
  batt_volts_V : Inport  Port=2
  spd_in_radps : Inport  Port=3
  Add : Sum  Inputs=|++
  Bus Selector : BusSelector  OutputSignals=powertrain.control.ctrl_eng_on,powertrain.signal4.batt_SoC_norm,vehicle.veh_spd_mps,powertrain.engine.eng_spd_radps,powertrain.engine.target_idle_spd_radps,driver.driver_brk_norm,powertrain.trans.ctrl.dct_core_ctrl.trans_curr_gear,powertrain.trans.ctrl.gear_num
  Compare To Constant2 : simulink/Logic and Bit Operations/Compare To Constant  relop=<=  const=alternator.regen_boost_max_battery_soc_norm  OutDataTypeStr=boolean  ZeroCross=off
  Compare To Zero{,1..3} (4 alike) : simulink/Logic and Bit Operations/Compare To Zero  relop=>  OutDataTypeStr=boolean  ZeroCross=off
  Constant2 : Constant  Value=alternator.regen_idle_speed_offset_radps
  Data Type Conversion : DataTypeConversion
  Divide : Product  Inputs=**//
  Input Output Elec Mech E&P Nm radps V A : Subsystem
  Lookup Table Dynamic : simulink/Lookup Tables/Lookup Table Dynamic  LookUpMeth=Interpolation-Use End Values  OutDataType=fixdt('double')  OutScaling=[]  OutputDataTypeScalingMode=Specify via dialog  OutDataTypeStr=fixdt('double')  DoSatur=off
  MinMax : MinMax  Function=max  Inputs=2
  MinMax1 : MinMax  Function=max  Inputs=2
  MinMax2 : MinMax  Function=max  Inputs=2
  Mux : Mux  Inputs=2
  Mux1 : Mux  Inputs=2
  PID Controller : simulink/Continuous/PID Controller  Controller=PID  TimeDomain=Continuous-time  SampleTime=-1  IntegratorMethod=Forward Euler  FilterMethod=Forward Euler  Form=Parallel  UseFilter=on  ControllerParametersSource=internal  P=alternator.nominal_Kp * (1 + alternator.regen_Kp_multiplier*alternator.regen_enable)  I=alternator.nominal_Ki * (1 + alternator.regen_Ki_multiplier*alternator.regen_enable)  D=0  N=1  InitialConditionSource=internal  InitialConditionForIntegrator=0  InitialConditionForFilter=0  ExternalReset=falling  ZeroCross=off  LimitOutput=on  UpperSaturationLimit=0  LowerSaturationLimit=-alternator.max_current_A  LinearizeAsGain=on  AntiWindupMode=clamping  Kb=1  TrackingMode=off  Kt=1  PParamMin=[]  PParamMax=[]  IParamMin=[]  IParamMax=[]  DParamMin=[]  DParamMax=[]  NParamMin=[]  NParamMax=[]  KbParamMin=[]  KbParamMax=[]  KtParamMin=[]  KtParamMax=[]  POutMin=[]  POutMax=[]  IOutMin=[]  IOutMax=[]  DOutMin=[]  DOutMax=[]  NOutMin=[]  NOutMax=[]  KbOutMin=[]  KbOutMax=[]  KtOutMin=[]  KtOutMax=[]  IntegratorOutMin=[]  IntegratorOutMax=[]  FilterOutMin=[]  FilterOutMax=[]  SumOutMin=[]  SumOutMax=[]  SumI1OutMin=[]  SumI1OutMax=[]  SumI2OutMin=[]  SumI2OutMax=[]  SumI3OutMin=[]  SumI3OutMax=[]  SumDOutMin=[]  SumDOutMax=[]  SaturationOutMin=[]  SaturationOutMax=[]  IntegratorContinuousStateAttributes=''  IntegratorStateMustResolveToSignalObject=off  IntegratorRTWStateStorageClass=Auto  FilterContinuousStateAttributes=''  FilterStateMustResolveToSignalObject=off  FilterRTWStateStorageClass=Auto  DifferentiatorICPrevScaledInput=0  DifferentiatorOutMin=[]  DifferentiatorOutMax=[]
  Product : Product
  Product1 : Product  Inputs=4
  Product2 : Product
  Product3 : Product
  Rate Limiter : RateLimiter  RisingSlewLimit=1/.15  FallingSlewLimit=-1/0.15
  Relational Operator : RelationalOperator  Operator=>  OutDataTypeStr=boolean  ZeroCross=off
  Relational Operator1 : RelationalOperator  OutDataTypeStr=boolean  ZeroCross=off
  Saturation : Saturate  UpperLimit=Inf  LowerLimit=eps
  Saturation2 : Saturate  UpperLimit=Inf  LowerLimit=1  ZeroCross=off
  Sum : Sum  Inputs=|+-
  Sum1 : Sum  Inputs=++|
  alternator state : Subsystem
  boost volts limit : Saturate  UpperLimit=alternator.regen_max_boost_volts  LowerLimit=0  ZeroCross=off
  brake boost gain : Gain  Gain=alternator.regen_max_boost_volts  OutDataTypeStr=double
  efficiency_norm : Constant  Value=alternator.efficiency_norm
  inertia_kgm2 : Constant  Value=alternator.inertia_kgm2
  regen enable : Gain  Gain=alternator.regen_enable
  sat : Saturate  UpperLimit=0.89  LowerLimit=0  ZeroCross=off
  target_voltage_V : Constant  Value=alternator.target_voltage_V
  target_voltage_V1 : Constant  Value=electric.battery.initial_soc_norm
  target_voltage_V2 : Constant  Value=0.9
  target_voltage_V3 : Constant
  target_voltage_V4 : Constant  Value=1 - alternator.regen_enable
  target_voltage_V5 : Constant  Value=electric.battery.min_voltage_V
  to datalog : Subsystem
  to datalog1 : Subsystem
  to datalog2 : Subsystem
  to datalog3 : Subsystem
  to datalog5 : Subsystem
  to datalog6 : Subsystem
  to datalog8 : Subsystem
  upshift boost volts : Gain  Gain=alternator.regen_upshift_boost_volts  OutDataTypeStr=double
  trq_out_Nm : Outport
  iner_out_kgm2 : Outport  Port=2
  curr_out_A : Outport  Port=3
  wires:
  sat/1 -> Mux/1
  Product3/1 -> upshift boost volts/1
  regen enable/1 -> Rate Limiter/1
  Rate Limiter/1 -> boost volts limit/1
  target_voltage_V5/1 -> MinMax2/2
  Product2/1 -> MinMax2/1
  MinMax1/1 -> Product2/1
  Data Type Conversion/1 -> MinMax1/2
  Compare To Zero3/1 -> Data Type Conversion/1
  MinMax2/1 -> Sum1/2
  Sum/1 -> PID Controller/1
  Product1/1 -> to datalog6/1(Var), Sum1/1, Compare To Zero3/1
  Mux1/1 -> Lookup Table Dynamic/3
  target_voltage_V4/1 -> Mux1/2
  target_voltage_V3/1 -> Mux1/1
  Mux/1 -> Lookup Table Dynamic/2
  target_voltage_V2/1 -> Mux/2
  target_voltage_V1/1 -> sat/1
  Compare To Zero2/1 -> brake boost gain/1
  Compare To Zero1/1 -> Product3/1
  Relational Operator/1 -> Product3/2
  upshift boost volts/1 -> MinMax/2, to datalog5/1(Var)
  Relational Operator1/1 -> Product1/3
  PID Controller/1 -> to datalog8/1(Var), Product/2
  MinMax/1 -> regen enable/1
  Bus Selector/7 -> Relational Operator/2, Compare To Zero1/1  "<trans_curr_gear>"
  Bus Selector/8 -> Relational Operator/1  "<gear_num>"
  Compare To Constant2/1 -> Product1/1
  system_bus/1 -> Bus Selector/1
  alternator state/1(state) -> Product/1, to datalog2/1(Var)
  Saturation2/1 -> Sum/1
  inertia_kgm2/1 -> Input Output Elec Mech E&P Nm radps V A/5(iner_out_kgm2), iner_out_kgm2/1
  Divide/1 -> trq_out_Nm/1, Input Output Elec Mech E&P Nm radps V A/3(trq_out_Nm)
  efficiency_norm/1 -> Divide/4
  Saturation/1 -> Divide/3
  spd_in_radps/1 -> Input Output Elec Mech E&P Nm radps V A/4(spd_out_radps), Saturation/1, alternator state/2(spd_in_radps)
  Product/1 -> Input Output Elec Mech E&P Nm radps V A/2(curr_in_A), curr_out_A/1, Divide/2
  target_voltage_V/1 -> Product2/2
  batt_volts_V/1 -> Saturation2/1, Input Output Elec Mech E&P Nm radps V A/1(volts_in_V), Divide/1
  Sum1/1 -> PID Controller/2, Sum/2, to datalog1/1(Var)
  Bus Selector/6 -> Compare To Zero2/1  "<driver_brk_norm>"
  brake boost gain/1 -> MinMax/1
  boost volts limit/1 -> Product1/4
  Bus Selector/3 -> Compare To Zero/1  "<veh_spd_mps>"
  Compare To Zero/1 -> Product1/2
  Bus Selector/2 -> Lookup Table Dynamic/1, Compare To Constant2/1  "<batt_SoC_norm>"
  Bus Selector/1 -> alternator state/1(eng_on)  "<ctrl_eng_on>"
  Lookup Table Dynamic/1 -> MinMax1/1, to datalog3/1(Var), to datalog/1(Var)
  Bus Selector/4 -> Relational Operator1/1  "<eng_spd_radps>"
  Add/1 -> Relational Operator1/2
  Bus Selector/5 -> Add/1  "<target_idle_spd_radps>"
  Constant2/1 -> Add/2

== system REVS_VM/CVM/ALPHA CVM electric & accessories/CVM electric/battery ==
  note: thermal model will eventually be a variant, probably, with a "simple" thermal model version
  system_bus : Inport
  curr_out_A : Inport  Port=2
  Bus Creator : BusCreator  Inputs=6
  Bus Selector : BusSelector  OutputSignals=temp_degC
  Elec E&P V A Standalone : Subsystem
  Gain : Gain  Gain=-1
  Memory2 : Memory
  battery power limits : Subsystem
  dynamic battery model : Subsystem
  thermal model : Subsystem
  bus_out : Outport
  volts_out_V : Outport  Port=2
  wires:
  Memory2/1 -> Bus Creator/5, dynamic battery model/2(curr_out_A)  "batt_curr_A"
  dynamic battery model/3(volts_out_V) -> Bus Creator/6, volts_out_V/1, Elec E&P V A Standalone/1(volts_V), battery power limits/4(volts_out_V)  "batt_volts_V"
  system_bus/1 -> Bus Selector/1
  dynamic battery model/6(loss_pwr_W) -> thermal model/1(loss_pwr_W)
  Gain/1 -> Elec E&P V A Standalone/2(curr_A)
  Bus Creator/1 -> bus_out/1
  curr_out_A/1 -> Memory2/1, Gain/1  "batt_curr_A"
  battery power limits/2(max_chg_pwr_W) -> Bus Creator/4  "batt_max_chg_pwr_W"
  battery power limits/1(max_dis_pwr_W) -> Bus Creator/3  "batt_max_dis_pwr_W"
  dynamic battery model/2(OCV_V) -> battery power limits/3(OCV_V)
  dynamic battery model/4(dis_res_Ohm) -> battery power limits/5(dis_res_Ohms)
  dynamic battery model/5(chg_res_Ohm) -> battery power limits/6(chg_res_Ohms)
  dynamic battery model/1(SoC_norm) -> battery power limits/2(SoC_norm), Bus Creator/2  "batt_SoC_norm"
  Bus Selector/1 -> thermal model/2(amb_temp_degC)  "<temp_degC>"
  thermal model/1(batt_temp_degC) -> dynamic battery model/1(batt_temp_degC), battery power limits/1(batt_temp_degC), Bus Creator/1  "batt_temp_degC"
